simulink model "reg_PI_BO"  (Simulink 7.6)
settings: Solver=ode15s  StartTime=0.0  StopTime=0.05  RelTol=1e-3
InitFcn:
  | clc, close all
  | Kp=1.02;
  | R1=10e3;
  | R2=(Kp-1)*R1;
  | 
  | Ti=0.01;
  | C2=Ti/(R1+R2);
libraries: fl_lib x8, nesl_utility x3, simulink x1, elec_lib x1

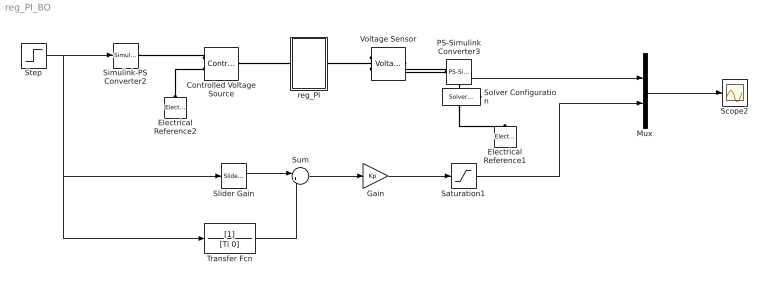
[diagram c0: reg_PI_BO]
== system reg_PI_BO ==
  Controlled Voltage Source : fl_lib/Electrical/Electrical Sources/Controlled Voltage Source  DialogController=NetworkEngine.DynNeDlgSource  SystemSampleTime=-1  i_Log=off  v_Log=off  LocalVarNames=|i|v  LocalVarDescs=|i|v  LocalVarLogging=[0 0]
  Electrical Reference1 : fl_lib/Electrical/Electrical Elements/Electrical Reference  DialogController=NetworkEngine.DynNeDlgSource  SystemSampleTime=-1  i_Log=off  LocalVarNames=|i  LocalVarDescs=|i  LocalVarLogging=[]
  Electrical Reference2 : fl_lib/Electrical/Electrical Elements/Electrical Reference  DialogController=NetworkEngine.DynNeDlgSource  SystemSampleTime=-1  i_Log=off  LocalVarNames=|i  LocalVarDescs=|i  LocalVarLogging=[]
  Gain : Gain  Gain=Kp
  Mux : Mux  Inputs=2
  PS-Simulink Converter3 : nesl_utility/PS-Simulink Converter  DialogController=NetworkEngine.DynNeUtilDlgSource  SystemSampleTime=-1  PhysicalDomain=network_engine_domain  LeftPortType=input  RightPortType=output  SubClassName=ps_output  Unit=V  AffineConversion=off
  Saturation1 : Saturate  UpperLimit=15  LowerLimit=-15
  Scope2 : Scope
  Simulink-PS Converter2 : nesl_utility/Simulink-PS Converter  DialogController=NetworkEngine.DynNeUtilDlgSource  SystemSampleTime=-1  PhysicalDomain=network_engine_domain  LeftPortType=input  RightPortType=output  SubClassName=ps_input  Unit=1  AffineConversion=off  InputFilterTimeConstant=.001  UdotUserProvided=0
  Slider Gain : simulink/Math Operations/Slider Gain  SystemSampleTime=-1  low=0  gain=1  high=2
  Solver Configuration : nesl_utility/Solver Configuration  DialogController=NetworkEngine.DynNeUtilDlgSource  SystemSampleTime=-1  PhysicalDomain=network_engine_domain  LeftPortType=input  RightPortType=generic  SubClassName=solver  Accelerate=off  Profile=off  ResidualTolerance=1e-9  MaxNonlinIter=12  MaxModeIter=2  DoFixedCost=off  UseLocalSampling=off  DoDC=off  LinearAlgebra=Sparse  LocalSolverSampleTime=.001  LocalSolverChoice=NE_BACKWARD_EULER_ADVANCER  UseLocalSolver=off
  Step : Step  Time=0.01  After=5  SampleTime=0
  Sum : Sum  Inputs=|++
  Transfer Fcn : TransferFcn  Denominator=[Ti 0]
  Voltage Sensor : fl_lib/Electrical/Electrical Sensors/Voltage Sensor  DialogController=NetworkEngine.DynNeDlgSource  SystemSampleTime=-1  i1_Log=off  v1_Log=off  LocalVarNames=|i1|v1  LocalVarDescs=|i1|v1  LocalVarLogging=[0 0]
  reg_PI : Subsystem
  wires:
  Step/1 -> Simulink-PS Converter2/1, Slider Gain/1, Transfer Fcn/1
  Mux/1 -> Scope2/1
  Slider Gain/1 -> Sum/1
  Sum/1 -> Gain/1
  Transfer Fcn/1 -> Sum/2
  Gain/1 -> Saturation1/1
  PS-Simulink Converter3/1 -> Mux/1
  Saturation1/1 -> Mux/2
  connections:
  Controlled Voltage Source/LConn1 -- reg_PI/LConn1
  Voltage Sensor/LConn1 -- reg_PI/RConn1
  Electrical Reference2/LConn1 -- Controlled Voltage Source/RConn2
  Controlled Voltage Source/RConn1 -- Simulink-PS Converter2/RConn1
  Voltage Sensor/RConn1 -- PS-Simulink Converter3/LConn1
  Voltage Sensor/RConn2 -- Solver Configuration/RConn1 -- Electrical Reference1/LConn1

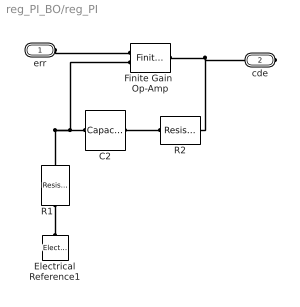
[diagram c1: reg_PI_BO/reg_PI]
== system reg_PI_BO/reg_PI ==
  C2 : fl_lib/Electrical/Electrical Elements/Capacitor  DialogController=NetworkEngine.DynNeDlgSource  SystemSampleTime=-1  c=C2 F  v0=0 V  r=1e-22 Ohm  g=0 1/Ohm  i_Log=off  v_Log=off  vc_Log=off  LocalVarNames=|i|v|vc  LocalVarDescs=|i|v|Internal variable for voltage across capacitor term  LocalVarLogging=[0 0 0]
  Electrical Reference1 : fl_lib/Electrical/Electrical Elements/Electrical Reference  DialogController=NetworkEngine.DynNeDlgSource  SystemSampleTime=-1  i_Log=off  LocalVarNames=|i  LocalVarDescs=|i  LocalVarLogging=[]
  Finite Gain  Op-Amp : elec_lib/Integrated Circuits/Finite Gain Op-Amp  DialogController=NetworkEngine.DynNeDlgSource  SystemSampleTime=-1  A=1000  Rin=1e+6 Ohm  Rout=100 Ohm  Vmin=-15 V  Vmax=15 V  LocalVarLogging=[]
  R1 : fl_lib/Electrical/Electrical Elements/Resistor  DialogController=NetworkEngine.DynNeDlgSource  SystemSampleTime=-1  R=R1 Ohm  i_Log=off  v_Log=off  LocalVarNames=|current|voltage|power  LocalVarDescs=|Resistor current (A)|Voltage across resistor (V)|Power (W)  LocalVarLogging=[0 0 0]
  R2 : fl_lib/Electrical/Electrical Elements/Resistor  DialogController=NetworkEngine.DynNeDlgSource  SystemSampleTime=-1  R=R2 Ohm  i_Log=off  v_Log=off  LocalVarNames=|current|voltage|power  LocalVarDescs=|Resistor current (A)|Voltage across resistor (V)|Power (W)  LocalVarLogging=[0 0 0]
  err : PMIOPort  Port=1  Side=Left
  cde : PMIOPort  Port=2  Side=Right
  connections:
  Finite Gain  Op-Amp/RConn1 -- cde/RConn1 -- R2/RConn1
  C2/LConn1 -- Finite Gain  Op-Amp/LConn2 -- R1/RConn1
  C2/RConn1 -- R2/LConn1
  R1/LConn1 -- Electrical Reference1/LConn1
  err/RConn1 -- Finite Gain  Op-Amp/LConn1
